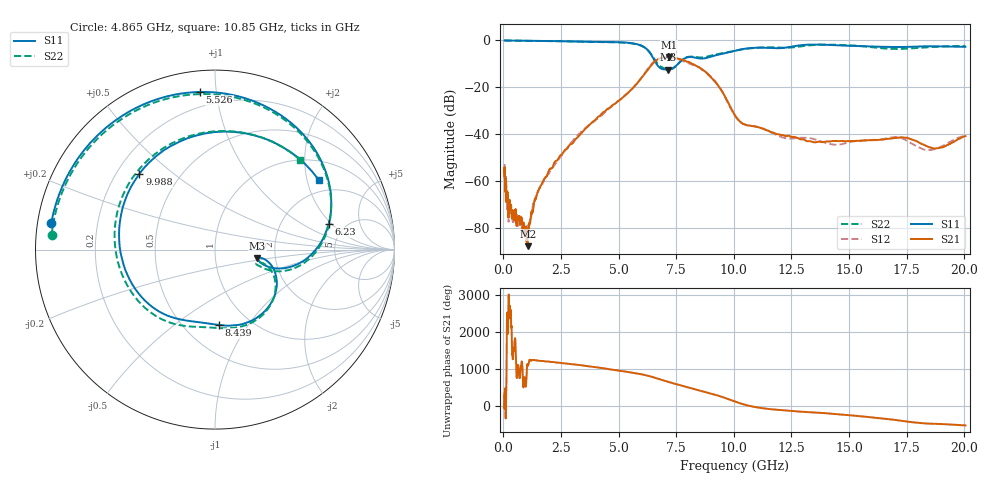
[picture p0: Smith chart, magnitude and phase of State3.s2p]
# Hz S DB R 50
!freq MagS11 AngS11 MagS21 AngS21 MagS12 AngS12 MagS22 AngS22
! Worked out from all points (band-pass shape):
!   1601 points, 50 MHz to 20.05 GHz, reference 50 ohm
!   highest |S21| = -7.04 dB at 7.183 GHz (marker M1); lowest = -87.6 dB at 1.055 GHz (marker M2)
!   |S21| within 3 dB of the highest: 6.463 GHz to 8.217 GHz (1.754 GHz wide, 23.9 % of centre)
!   lowest |S11| = -12.4 dB at 7.13 GHz (marker M3), VSWR 1.63, Z = 80.2 - j8.12 ohm
!   |S11| at or under -10 dB: 6.645 GHz to 7.571 GHz (926 MHz wide, 13 % of centre)
!   |S22| runs from -12.3 to 0.0 dB; largest |S21 - S12| = 0.029
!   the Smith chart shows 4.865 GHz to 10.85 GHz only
!   S11 on the Smith chart (normalised r, x): 4.865 GHz: 0.04, +0.08; 5.526 GHz: 0.11, +0.90; 6.23 GHz: 3.74, +1.84; 8.439 GHz: 0.72, -0.74; 9.988 GHz: 0.29, +0.38; 10.85 GHz: 1.56, +2.36
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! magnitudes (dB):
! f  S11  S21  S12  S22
! 50 MHz  0.0  -56.4  -52.6  0.0
! 81.68 MHz  0.0  -59.6  -63.8  0.0
! 89.7 MHz  0.0  -62.8  -58.5  0.0
! 100.7 MHz  0.0  -60.7  -67.7  0.0
! 110.2 MHz  0.0  -66.9  -60.1  0.0
! 135.9 MHz  0.0  -65.1  -65.8  0.0
! 224.6 MHz  0.0  -73.3  -76.8  0.0
! 369.6 MHz  0.0  -74.6  -74.0  0.0
! 1.005 GHz  -0.1  -84.9  -79.9  -0.1
! 1.055 GHz  -0.1  -87.6  -79.9  -0.1
! 2.722 GHz  -0.3  -46.3  -46.2  -0.4
! 4.865 GHz  -0.7  -26.7  -26.7  -0.8
! 5.526 GHz  -1.1  -21.1  -21.2  -1.2
! 6.23 GHz  -3.8  -13.0  -12.5  -3.8
! 7.13 GHz  -12.4  -7.0  -7.1  -12.2
! 7.183 GHz  -12.4  -7.0  -7.1  -12.3
! 7.402 GHz  -11.5  -7.3  -7.5  -11.6
! 8.439 GHz  -7.5  -11.1  -11.2  -7.2
! 9.988 GHz  -4.5  -30.9  -31.1  -4.5
! 10.85 GHz  -3.1  -36.5  -36.4  -3.2
! 18.39 GHz  -2.4  -45.2  -46.7  -2.9
! 20.05 GHz  -2.7  -40.7  -40.5  -2.3
